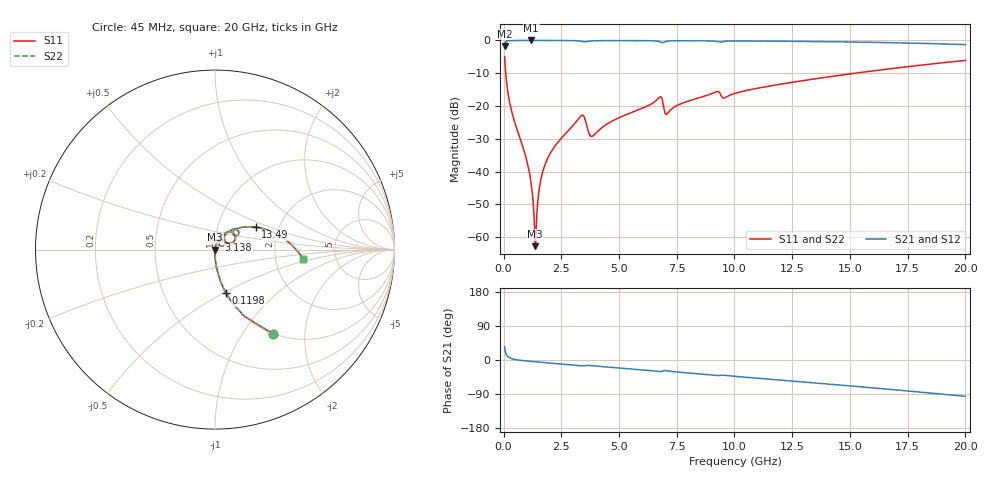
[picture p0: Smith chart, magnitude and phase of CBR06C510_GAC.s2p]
! S-parameter model data by Modelithics Inc.  support@modelithics.com 813-866-6335  Tampa FL USA
! S-Parameter data specifications:
! Substrate: 20-mil Rogers 4350B, substrate thickness, H=0.508mm, Dielectric constant, Er=3.75
! PCB Mounting Pad Footprint: Pad width, PadW=0.85mm , Pad length, PadL=0.64mm , Pad gap, PadG (edge-to-edge)=0.62mm , Reference planes=1.9mm apart
#  GHz  S  MA  R 50
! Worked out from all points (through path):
!   801 points, 45 MHz to 20 GHz, reference 50 ohm
!   highest |S21| = -0.01 dB at 1.192 GHz (marker M1); lowest = -1.7 dB at 45 MHz (marker M2)
!   group delay of S21, straight-line fit = 13.5 ps
!   lowest |S11| = -62.8 dB at 1.367 GHz (marker M3), VSWR 1.00, Z = 50.1 - j0.0386 ohm
!   |S11| at or under -10 dB: 93.09 MHz to 15.23 GHz (15.13 GHz wide, 198 % of centre)
!   |S22| runs from -62.8 to -4.9 dB; largest |S21 - S12| = 0
!   S11 on the Smith chart (normalised r, x): 45 MHz: 1.00, -1.38; 119.8 MHz: 1.00, -0.51; 3.138 GHz: 1.04, +0.11; 13.49 GHz: 1.52, +0.41; 20 GHz: 2.90, -0.41
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0.045  0.5681 -55.5  0.8226 34.5  0.8226 34.5  0.5681 -55.5
0.119831  0.2495 -75.9  0.9681 14.0  0.9681 14.0  0.2495 -75.9
0.319381  0.09187 -85.6  0.9954 4.2  0.9954 4.2  0.09187 -85.6
0.967919  0.01645 -90.5  0.9993 -2.4  0.9993 -2.4  0.01645 -90.5
1.192413  0.006668 -88.5  0.9993 -3.7  0.9993 -3.7  0.006668 -88.5
1.292188  0.003 -82.2  0.9993 -4.3  0.9993 -4.3  0.003 -82.2
1.367019  0.000727 -32.0  0.9993 -4.7  0.9993 -4.7  0.000727 -32.0
1.44185  0.002242 67.6  0.9993 -5.1  0.9993 -5.1  0.002242 67.6
1.616456  0.007577 78.6  0.9992 -6.0  0.9992 -6.0  0.007577 78.6
1.865894  0.01469 79.6  0.999 -7.3  0.999 -7.3  0.01469 79.6
3.138025  0.05726 67.5  0.9899 -14.1  0.9899 -14.1  0.05726 67.5
3.387462  0.07228 48.5  0.9659 -15.4  0.9659 -15.4  0.07228 48.5
3.83645  0.03453 46.7  0.983 -15.0  0.983 -15.0  0.03453 46.7
6.704981  0.1306 49.8  0.9692 -30.4  0.9692 -30.4  0.1306 49.8
7.079137  0.07571 44.0  0.9742 -28.4  0.9742 -28.4  0.07571 44.0
9.199356  0.1643 43.2  0.9688 -40.8  0.9688 -40.8  0.1643 43.2
9.548569  0.1322 39.9  0.968 -40.0  0.968 -40.0  0.1322 39.9
10.0225  0.1558 45.0  0.9821 -43.1  0.9821 -43.1  0.1558 45.0
13.36496  0.2559 29.4  0.9631 -59.9  0.9631 -59.9  0.2559 29.4
13.48968  0.2597 28.8  0.962 -60.6  0.962 -60.6  0.2597 28.8
16.68248  0.3676 12.2  0.9258 -77.3  0.9258 -77.3  0.3676 12.2
20  0.4957 -6.2  0.8636 -95.8  0.8636 -95.8  0.4957 -6.2
